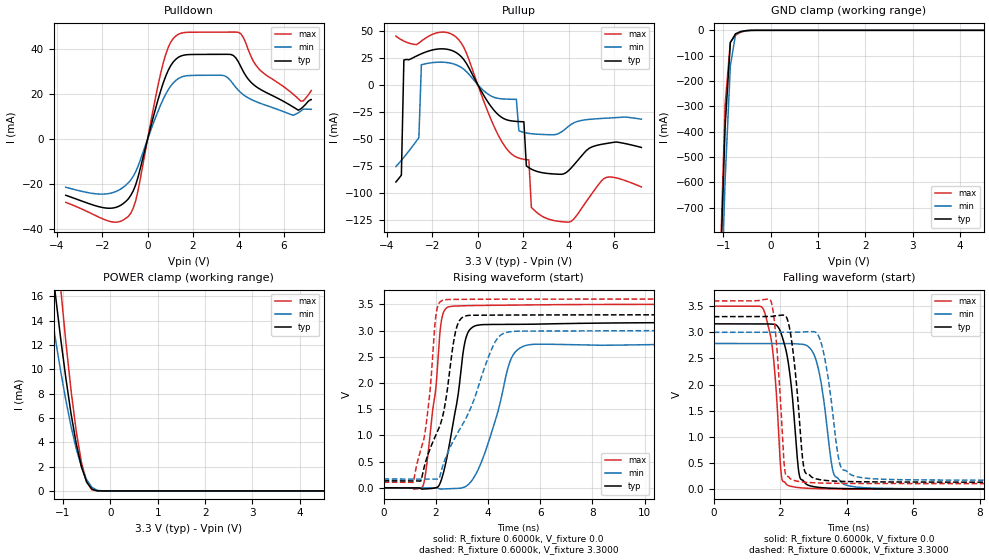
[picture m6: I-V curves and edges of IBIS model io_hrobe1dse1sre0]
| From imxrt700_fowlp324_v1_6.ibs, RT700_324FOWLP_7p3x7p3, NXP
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[Model] io_hrobe1dse1sre0
|   Model io_hrobe1dse1sre0
| This model was characterised for following simulation conditions:
| External (pad) voltage:
|   - Typ: 3.3V,   - Min: 3.0V,   - Max: 3.6V
| Library cells for typ/min/max conditions are connected as defined below:
|  PAD_IO - External Pad
|  ipp_do - Core Input
|  ipp_obe - Output Buffer Enable
|  ASRCN3V3[3] - NC
|  ASRCN3V3[4] - NC
|  ASRCP3V3[4] - NC
|  REFAPBIAS3V3 - gnde
|  REFBAMPL3V3 - vdd1v8
|  REFCAMPH3V3 - vdd1v8
|  REFDNBIAS3V3 - vdd1v8
|  REFH3V3 - REFH3V3
|  REFL3V3 - REFL3V3
|  gnde - gnde
|  ipp_dse - vdd
|  ipp_ina235_3v - NC
|  ipp_ina40_3v - NC
|  ipp_ina_mux - NC
|  ipp_ind - NC
|  ipp_ind_1p8v - NC
|  ipp_ind_3v - NC
|  ipp_sre - gnde
|  vdd - vdd
|  vdd1v8 - vdd1v8
|  vdda - vdde3v3
|  vdde3v3 - vdde3v3
| All other pins connected to ground
Model_type I/O
Polarity   Non-Inverting
Enable   Active-High
Vinl =   0.9900V
Vinh =   2.3100V
Vmeas =  1.6500V
Cref =   15.0000pF
Rref =   0.6000k
Vref =   0.0V
C_comp   4.0008pF   3.8189pF   4.1206pF
|C_comp_pullup   0.5645pF   0.7342pF   0.4704pF
|C_comp_pulldown   2.1154pF   2.2136pF   1.8991pF
[Model Spec]
| variable   typ   min   max
Vinh   2.3100V   NA   NA
Vinl   0.9900V   NA   NA
Vref   0.0V   0.0V   0.0V
Cref   15.0000pF   15.0000pF   15.0000pF
Rref   0.6000k   0.6000k   0.6000k
[Receiver Thresholds]
Vcross_high  =   0.0V
Vcross_low  =   0.0V
Vdiff_ac  =   0.0V
Vdiff_dc  =   0.0V
Tdiffslew_ac  =   0.0S
[Temperature Range]   25.0000   0.1250k   -40.0000
[Voltage Range]   3.3000V   3.0000V   3.6000V
[Pullup Reference]   3.3000V   3.0000V   3.6000V
[Pulldown Reference]   0.0V   0.0V   0.0V
[POWER Clamp Reference]   3.3000V   3.0000V   3.6000V
[GND Clamp Reference]   0.0V   0.0V   0.0V
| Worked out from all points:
|   slope of the pulldown table from 0 to 0.495 V, typ, clamps not added: 26.5 ohm
|   slope of the pullup table from 0 to 0.495 V, typ, clamps not added: 28.3 ohm
|   GND clamp passes 1 mA (typ) near -0.49 V on its own axis
|   POWER clamp passes 1 mA (typ) near -0.52 V on its own axis
|   rising waveform, R_fixture 0.6000k, V_fixture 0.0: 20-80 % time 584ps typ, 933ps min, 416ps max; typ from 0 V to 3.16 V
|   rising waveform, R_fixture 0.6000k, V_fixture 3.3000: 20-80 % time 848ps typ, 1.46ns min, 456ps max; typ from 0.133 V to 3.3 V
|   falling waveform, R_fixture 0.6000k, V_fixture 0.0: 20-80 % time 295ps typ, 356ps min, 240ps max; typ from 3.16 V to 0 V
|   falling waveform, R_fixture 0.6000k, V_fixture 3.3000: 20-80 % time 266ps typ, 357ps min, 211ps max; typ from 3.3 V to 0.133 V
[Pulldown]
|Voltage   I(typ)   I(min)   I(max)
-3.6V     -24.95mA   -21.38mA   -28.1mA
-1.73V    -30.7mA    -24.22mA   -36.35mA
-740mV    -24.98mA   -18.14mA   -32.92mA
-410mV    -16.5mA    -11.78mA   -22.36mA
690mV     24.99mA    17.78mA    33.89mA
1.02V     32.66mA    23.61mA    43.07mA
1.35V     36.31mA    26.85mA    46.53mA
3.33V     37.63mA    28.24mA    47.5mA
3.99V     34.37mA    21.72mA    47.42mA
5.09V     21.35mA    15.41mA    29.39mA
6.74V     13.43mA    12.45mA    16.89mA
7.2V      17.54mA    13.21mA    21.56mA
[Pullup]
|Voltage   I(typ)   I(min)   I(max)
-3.6V     -89.83mA   -75.63mA   44.86mA
-3.36V    -83.54mA   -69.87mA   41.48mA
-3.25V    22.81mA    -67.08mA   40.27mA
-2.59V    27.52mA    -48.89mA   38.49mA
-2.48V    28.55mA    18.37mA    40.31mA
-1.82V    32.75mA    20.69mA    47.77mA
1.7V      -33.91mA   -13.55mA   -66.88mA
2.03V     -34.28mA   -44.12mA   -68.87mA
2.25V     -76.64mA   -45.01mA   -69.46mA
2.36V     -77.99mA   -45.29mA   -113.3mA
2.69V     -80.62mA   -45.82mA   -119.5mA
7.2V      -57.95mA   -31.85mA   -94.39mA
[GND_clamp]
|Voltage   I(typ)   I(min)   I(max)
-3.6V     -19.67A    -19.55A    -20.65A
-1.07V    -1.013A    -1.224A    -956.3mA
-960mV    -377.1mA   -587.4mA   -291.7mA
-850mV    -48.21mA   -140.8mA   -46.94mA
-740mV    -13.57mA   -15.59mA   -19.22mA
-630mV    -5.137mA   -4.351mA   -7.235mA
-520mV    -1.276mA   -1.53mA    -1.554mA
-300mV    -4.403uA   -32.47uA   -997nA
7.2V      0A         0A         0A
[POWER_clamp]
|Voltage   I(typ)   I(min)   I(max)
-3.6V     102.5mA    81.21mA    131.1mA
-1.38V    23.81mA    18.18mA    31.78mA
-1.27V    19.88mA    15.26mA    26.56mA
-1.16V    16.12mA    12.48mA    21.52mA
-1.05V    12.56mA    9.868mA    16.71mA
-830mV    6.344mA    5.304mA    8.253mA
-720mV    3.878mA    3.458mA    4.888mA
-610mV    1.973mA    1.979mA    2.327mA
-500mV    725uA      918.2uA    733.4uA
-390mV    144.3uA    301.5uA    95.95uA
-170mV    198.2nA    4.056uA    20.28nA
7.2V      0A         0A         0A
[Ramp]
| variable   typ   min   max
dV/dt_r  1.8972/0.5839n   1.6717/0.9333n   2.1003/0.4159n
dV/dt_f  1.9001/0.2655n   1.6991/0.3570n   2.0958/0.2106n
R_load = 0.6000k
[Rising Waveform]
R_fixture= 0.6000k
V_fixture= 0.0
V_fixture_min= 0.0
V_fixture_max= 0.0
|time   V(typ)   V(min)   V(max)
0s        75.99nV    1.221uV    58.53nV
1.521ns   -23.7mV    -450.8uV   52.9mV
2ns       1.549mV    -2.311mV   1.895V
2.213ns   153.3mV    -23.45mV   3.185V
2.628ns   1.134V     -16.88mV   3.463V
3.301ns   3.015V     89.77mV    3.475V
4.001ns   3.115V     841mV      3.48V
4.875ns   3.118V     2.448V     3.487V
5.664ns   3.12V      2.733V     3.491V
60ns      3.162V     2.786V     3.5V
[Rising Waveform]
R_fixture= 0.6000k
V_fixture= 3.3000
V_fixture_min= 3.0000
V_fixture_max= 3.6000
|time   V(typ)   V(min)   V(max)
0s        133.2mV    168.1mV    107mV
1.14ns    132.6mV    168.1mV    110.1mV
1.608ns   493.4mV    168mV      1.125V
2.034ns   1.043V     165.9mV    3.383V
2.334ns   1.538V     517.5mV    3.585V
2.705ns   2.853V     929.3mV    3.593V
2.923ns   3.2V       1.12V      3.595V
4.242ns   3.294V     2.753V     3.598V
4.879ns   3.296V     2.98V      3.599V
60ns      3.3V       3V         3.6V
[Falling Waveform]
R_fixture= 0.6000k
V_fixture= 0.0
V_fixture_min= 0.0
V_fixture_max= 0.0
|time   V(typ)   V(min)   V(max)
0s        3.162V     2.786V     3.5V
1.5ns     3.163V     2.786V     3.432V
1.775ns   3.157V     2.785V     2.643V
1.961ns   3.076V     2.788V     962.9mV
2.063ns   2.91V      2.788V     169.7mV
2.624ns   187.3mV    2.774V     25.19mV
3.13ns    36.44mV    2.35V      9.717mV
3.627ns   16.11mV    269.6mV    4.662mV
4.41ns    7.07mV     32.94mV    1.812mV
60ns      363.4nV    1.163uV    276nV
[Falling Waveform]
R_fixture= 0.6000k
V_fixture= 3.3000
V_fixture_min= 3.0000
V_fixture_max= 3.6000
|time   V(typ)   V(min)   V(max)
0s        3.3V       3V         3.6V
1.717ns   3.303V     3V         3.601V
1.878ns   3.316V     2.999V     2.859V
2.184ns   3.295V     3.001V     250.6mV
2.403ns   2.54V      3.001V     169mV
2.744ns   332.4mV    3.009V     132.4mV
3.247ns   175.9mV    2.764V     116.7mV
3.824ns   149.3mV    426.9mV    111.1mV
4.663ns   139.8mV    204.6mV    108.5mV
60ns      133.2mV    168.1mV    107mV
